PROGRAM P_Prog2
VAR

	fbKL6401 					: FB_LON_KL6401;

	fbREAD_032		: FB_READ_032_SNVT_res_kilo;
	fbSEND_032		: FB_SEND_032_SNVT_res_kilo;

	fbREAD_033		: FB_READ_033_SNVT_sound_db;
	fbSEND_033		: FB_SEND_033_SNVT_sound_db;

	fbREAD_034		: FB_READ_034_SNVT_speed;
	fbSEND_034		: FB_SEND_034_SNVT_speed;

	fbREAD_035		: FB_READ_035_SNVT_speed_mil;
	fbSEND_035		: FB_SEND_035_SNVT_speed_mil;

	fbREAD_036		: FB_READ_036_SNVT_str_asc;
	fbSEND_036		: FB_SEND_036_SNVT_str_asc;

	fbREAD_037		: FB_READ_037_SNVT_str_int;
	fbSEND_037		: FB_SEND_037_SNVT_str_int;

	fbREAD_038		: FB_READ_038_SNVT_telcom;
	fbSEND_038		: FB_SEND_038_SNVT_telcom;

	fbREAD_039		: FB_READ_039_SNVT_temp;
	fbSEND_039		: FB_SEND_039_SNVT_temp;
(*
	fbREAD_040		: FB_READ_040;
	fbSEND_040		: FB_SEND_008_SNVT_count;
*)
	fbREAD_041		: FB_READ_041_SNVT_vol;
	fbSEND_041		: FB_SEND_041_SNVT_vol;

	fbREAD_042		: FB_READ_042_SNVT_vol_kilo;
	fbSEND_042		: FB_SEND_042_SNVT_vol_kilo;

	fbREAD_043		: FB_READ_043_SNVT_vol_mil;
	fbSEND_043		: FB_SEND_043_SNVT_vol_mil;

	fbREAD_044		: FB_READ_044_SNVT_volt;
	fbSEND_044		: FB_SEND_044_SNVT_volt;

	fbREAD_045		: FB_READ_045_SNVT_volt_dbmv;
	fbSEND_045		: FB_SEND_045_SNVT_volt_dbmv;

	fbREAD_046		: FB_READ_046_SNVT_volt_kilo;
	fbSEND_046		: FB_SEND_046_SNVT_volt_kilo;

	fbREAD_047		: FB_READ_047_SNVT_volt_mil;
	fbSEND_047		: FB_SEND_047_SNVT_volt_mil;

	fbREAD_048		: FB_READ_048_SNVT_amp_f;
	fbSEND_048		: FB_SEND_048_SNVT_amp_f;

	fbREAD_049		: FB_READ_049_SNVT_angle_f;
	fbSEND_049		: FB_SEND_049_SNVT_angle_f;

	fbREAD_050		: FB_READ_050_SNVT_angle_vel_f;
	fbSEND_050		: FB_SEND_050_SNVT_angle_vel_f;

	fbREAD_051		: FB_READ_051_SNVT_count_f;
	fbSEND_051		: FB_SEND_051_SNVT_count_f;

	fbREAD_052		: FB_READ_052_SNVT_count_inc_f;
	fbSEND_052		: FB_SEND_052_SNVT_count_inc_f;

	fbREAD_053		: FB_READ_053_SNVT_flow_f;
	fbSEND_053		: FB_SEND_053_SNVT_flow_f;

	fbREAD_054		: FB_READ_054_SNVT_length_f;
	fbSEND_054		: FB_SEND_054_SNVT_length_f;

	fbREAD_055		: FB_READ_055_SNVT_lev_cont_f;
	fbSEND_055		: FB_SEND_055_SNVT_lev_cont_f;

	fbREAD_056		: FB_READ_056_SNVT_mass_f;
	fbSEND_056		: FB_SEND_056_SNVT_mass_f;

	fbREAD_057		: FB_READ_057_SNVT_power_f;
	fbSEND_057		: FB_SEND_057_SNVT_power_f;

	fbREAD_058		: FB_READ_058_SNVT_ppm_f;
	fbSEND_058		: FB_SEND_058_SNVT_ppm_f;

	fbREAD_059		: FB_READ_059_SNVT_press_f;
	fbSEND_059		: FB_SEND_059_SNVT_press_f;

	fbREAD_060		: FB_READ_060_SNVT_res_f;
	fbSEND_060		: FB_SEND_060_SNVT_res_f;

	fbREAD_061		: FB_READ_061_SNVT_sound_db_f;
	fbSEND_061		: FB_SEND_061_SNVT_sound_db_f;

	fbREAD_062		: FB_READ_062_SNVT_speed_f;
	fbSEND_062		: FB_SEND_062_SNVT_speed_f;

END_VAR

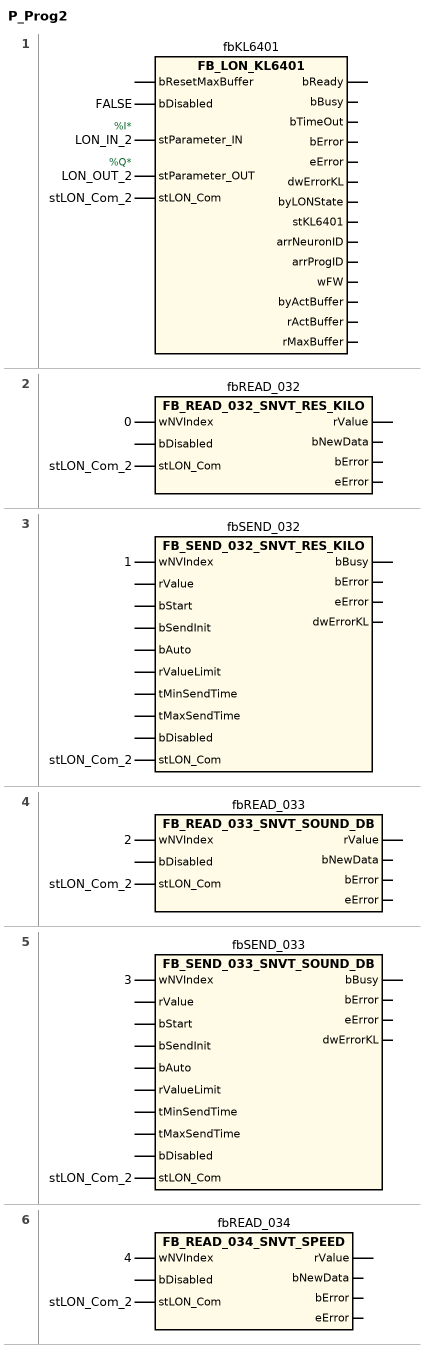
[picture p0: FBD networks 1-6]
// NETWORK 1
//   LON_IN_2: AT %I*
//   LON_OUT_2: AT %Q*
fbKL6401(
    bDisabled := FALSE,
    stParameter_IN := LON_IN_2,
    stParameter_OUT := LON_OUT_2,
    stLON_Com := stLON_Com_2); // FB_LON_KL6401

// NETWORK 2
fbREAD_032(wNVIndex := 0, stLON_Com := stLON_Com_2); // FB_READ_032_SNVT_RES_KILO

// NETWORK 3
fbSEND_032(wNVIndex := 1, stLON_Com := stLON_Com_2); // FB_SEND_032_SNVT_RES_KILO

// NETWORK 4
fbREAD_033(wNVIndex := 2, stLON_Com := stLON_Com_2); // FB_READ_033_SNVT_SOUND_DB

// NETWORK 5
fbSEND_033(wNVIndex := 3, stLON_Com := stLON_Com_2); // FB_SEND_033_SNVT_SOUND_DB

// NETWORK 6
fbREAD_034(wNVIndex := 4, stLON_Com := stLON_Com_2); // FB_READ_034_SNVT_SPEED

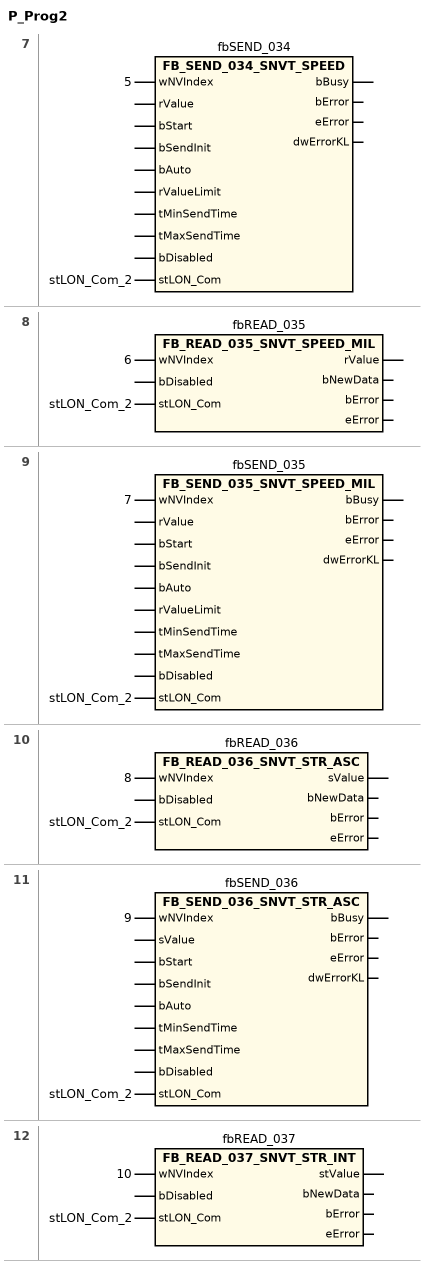
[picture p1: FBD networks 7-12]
// NETWORK 7
fbSEND_034(wNVIndex := 5, stLON_Com := stLON_Com_2); // FB_SEND_034_SNVT_SPEED

// NETWORK 8
fbREAD_035(wNVIndex := 6, stLON_Com := stLON_Com_2); // FB_READ_035_SNVT_SPEED_MIL

// NETWORK 9
fbSEND_035(wNVIndex := 7, stLON_Com := stLON_Com_2); // FB_SEND_035_SNVT_SPEED_MIL

// NETWORK 10
fbREAD_036(wNVIndex := 8, stLON_Com := stLON_Com_2); // FB_READ_036_SNVT_STR_ASC

// NETWORK 11
fbSEND_036(wNVIndex := 9, stLON_Com := stLON_Com_2); // FB_SEND_036_SNVT_STR_ASC

// NETWORK 12
fbREAD_037(wNVIndex := 10, stLON_Com := stLON_Com_2); // FB_READ_037_SNVT_STR_INT

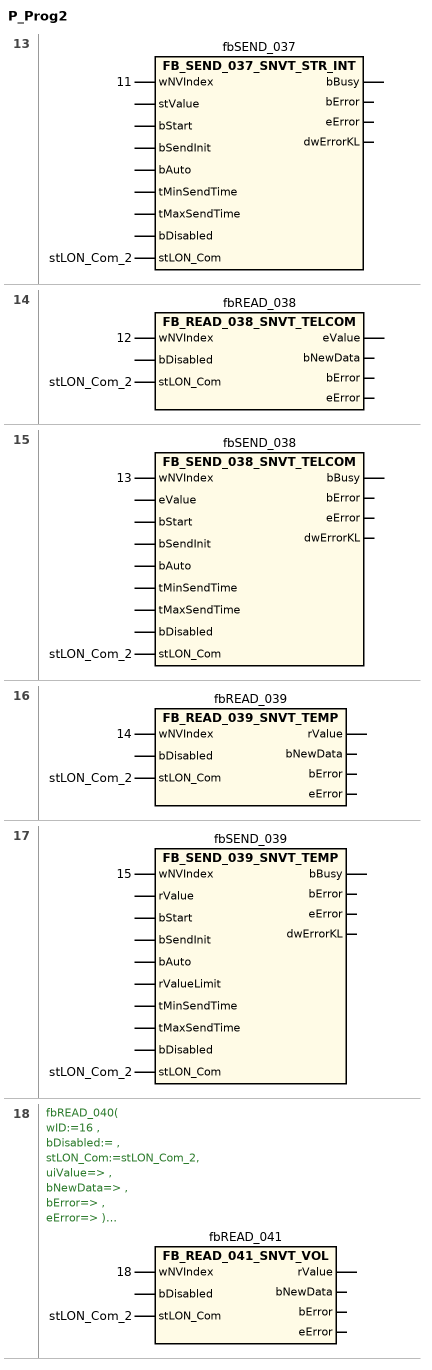
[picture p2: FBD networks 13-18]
// NETWORK 13
fbSEND_037(wNVIndex := 11, stLON_Com := stLON_Com_2); // FB_SEND_037_SNVT_STR_INT

// NETWORK 14
fbREAD_038(wNVIndex := 12, stLON_Com := stLON_Com_2); // FB_READ_038_SNVT_TELCOM

// NETWORK 15
fbSEND_038(wNVIndex := 13, stLON_Com := stLON_Com_2); // FB_SEND_038_SNVT_TELCOM

// NETWORK 16
fbREAD_039(wNVIndex := 14, stLON_Com := stLON_Com_2); // FB_READ_039_SNVT_TEMP

// NETWORK 17
fbSEND_039(wNVIndex := 15, stLON_Com := stLON_Com_2); // FB_SEND_039_SNVT_TEMP

// NETWORK 18
//
//
// fbREAD_040(
// 	wID:=16 ,
// 	bDisabled:= ,
// 	stLON_Com:=stLON_Com_2,
// 	uiValue=> ,
// 	bNewData=> ,
// 	bError=> ,
// 	eError=> );
// fbREAD_040.uiValue;
// fbREAD_040.bError;
// fbREAD_040.eError;
//
// fbSEND_040(
// 	wID:=17 ,
// 	bStart:= ,
// 	uiValue:= ,
// 	bDisabled:= ,
// 	stLON_Com:=stLON_Com_2,
// 	bError=> ,
// 	eError=> );
// fbSEND_040.uiValue;
// fbSEND_040.bStart;
// fbSEND_040.bError;
// fbSEND_040.eError;
//
//
//
//   fbREAD_041: fbREAD_040 : FB_READ_040; fbSEND_040 : FB_SEND_008_SNVT_count;
fbREAD_041(wNVIndex := 18, stLON_Com := stLON_Com_2); // FB_READ_041_SNVT_VOL

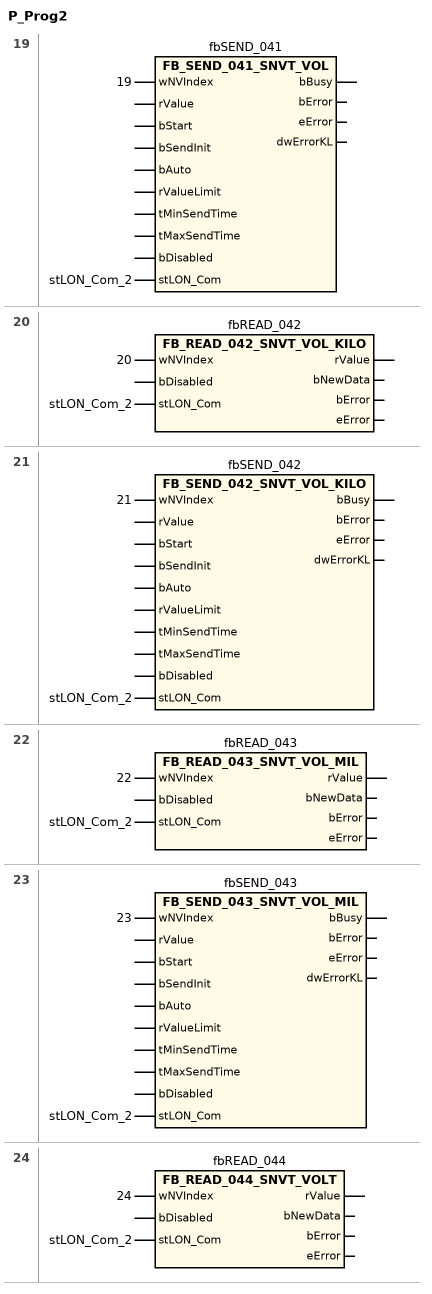
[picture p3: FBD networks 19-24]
// NETWORK 19
fbSEND_041(wNVIndex := 19, stLON_Com := stLON_Com_2); // FB_SEND_041_SNVT_VOL

// NETWORK 20
fbREAD_042(wNVIndex := 20, stLON_Com := stLON_Com_2); // FB_READ_042_SNVT_VOL_KILO

// NETWORK 21
fbSEND_042(wNVIndex := 21, stLON_Com := stLON_Com_2); // FB_SEND_042_SNVT_VOL_KILO

// NETWORK 22
fbREAD_043(wNVIndex := 22, stLON_Com := stLON_Com_2); // FB_READ_043_SNVT_VOL_MIL

// NETWORK 23
fbSEND_043(wNVIndex := 23, stLON_Com := stLON_Com_2); // FB_SEND_043_SNVT_VOL_MIL

// NETWORK 24
fbREAD_044(wNVIndex := 24, stLON_Com := stLON_Com_2); // FB_READ_044_SNVT_VOLT

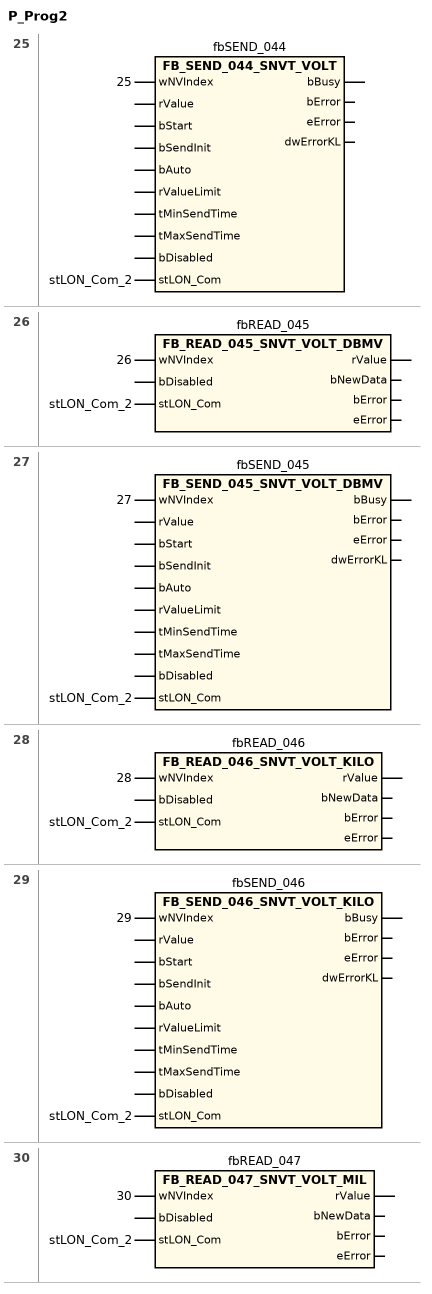
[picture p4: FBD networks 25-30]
// NETWORK 25
fbSEND_044(wNVIndex := 25, stLON_Com := stLON_Com_2); // FB_SEND_044_SNVT_VOLT

// NETWORK 26
fbREAD_045(wNVIndex := 26, stLON_Com := stLON_Com_2); // FB_READ_045_SNVT_VOLT_DBMV

// NETWORK 27
fbSEND_045(wNVIndex := 27, stLON_Com := stLON_Com_2); // FB_SEND_045_SNVT_VOLT_DBMV

// NETWORK 28
fbREAD_046(wNVIndex := 28, stLON_Com := stLON_Com_2); // FB_READ_046_SNVT_VOLT_KILO

// NETWORK 29
fbSEND_046(wNVIndex := 29, stLON_Com := stLON_Com_2); // FB_SEND_046_SNVT_VOLT_KILO

// NETWORK 30
fbREAD_047(wNVIndex := 30, stLON_Com := stLON_Com_2); // FB_READ_047_SNVT_VOLT_MIL

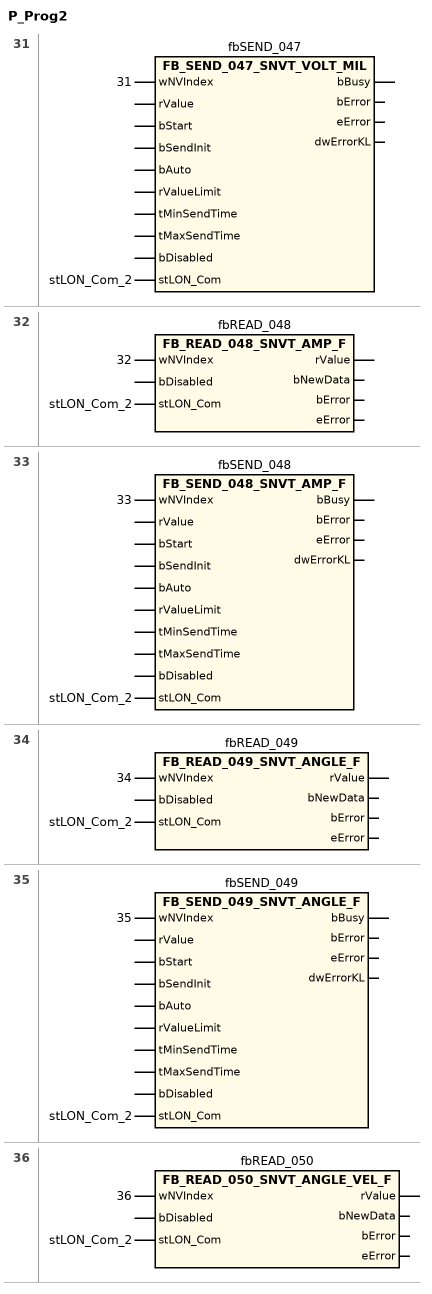
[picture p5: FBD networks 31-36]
// NETWORK 31
fbSEND_047(wNVIndex := 31, stLON_Com := stLON_Com_2); // FB_SEND_047_SNVT_VOLT_MIL

// NETWORK 32
fbREAD_048(wNVIndex := 32, stLON_Com := stLON_Com_2); // FB_READ_048_SNVT_AMP_F

// NETWORK 33
fbSEND_048(wNVIndex := 33, stLON_Com := stLON_Com_2); // FB_SEND_048_SNVT_AMP_F

// NETWORK 34
fbREAD_049(wNVIndex := 34, stLON_Com := stLON_Com_2); // FB_READ_049_SNVT_ANGLE_F

// NETWORK 35
fbSEND_049(wNVIndex := 35, stLON_Com := stLON_Com_2); // FB_SEND_049_SNVT_ANGLE_F

// NETWORK 36
fbREAD_050(wNVIndex := 36, stLON_Com := stLON_Com_2); // FB_READ_050_SNVT_ANGLE_VEL_F

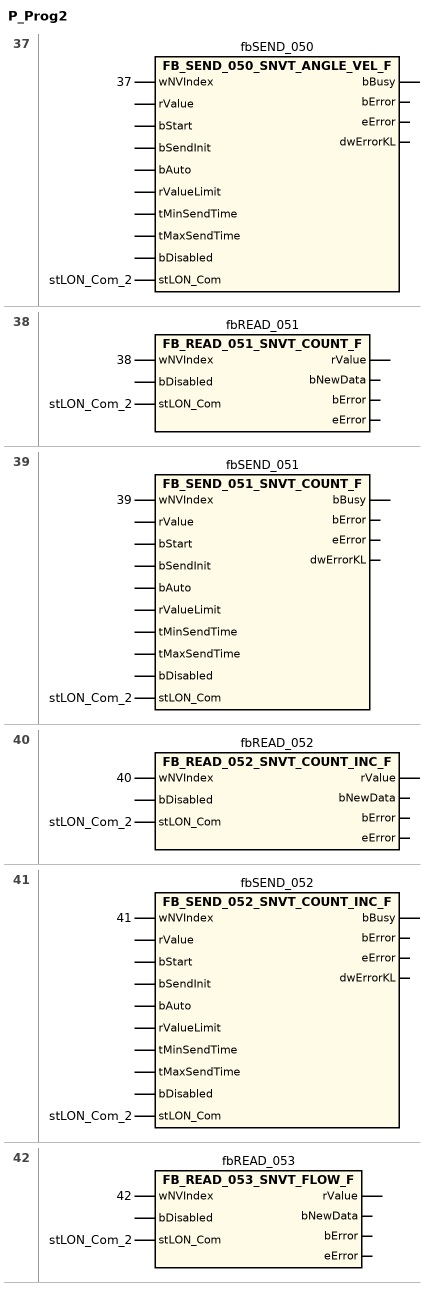
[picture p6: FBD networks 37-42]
// NETWORK 37
fbSEND_050(wNVIndex := 37, stLON_Com := stLON_Com_2); // FB_SEND_050_SNVT_ANGLE_VEL_F

// NETWORK 38
fbREAD_051(wNVIndex := 38, stLON_Com := stLON_Com_2); // FB_READ_051_SNVT_COUNT_F

// NETWORK 39
fbSEND_051(wNVIndex := 39, stLON_Com := stLON_Com_2); // FB_SEND_051_SNVT_COUNT_F

// NETWORK 40
fbREAD_052(wNVIndex := 40, stLON_Com := stLON_Com_2); // FB_READ_052_SNVT_COUNT_INC_F

// NETWORK 41
fbSEND_052(wNVIndex := 41, stLON_Com := stLON_Com_2); // FB_SEND_052_SNVT_COUNT_INC_F

// NETWORK 42
fbREAD_053(wNVIndex := 42, stLON_Com := stLON_Com_2); // FB_READ_053_SNVT_FLOW_F

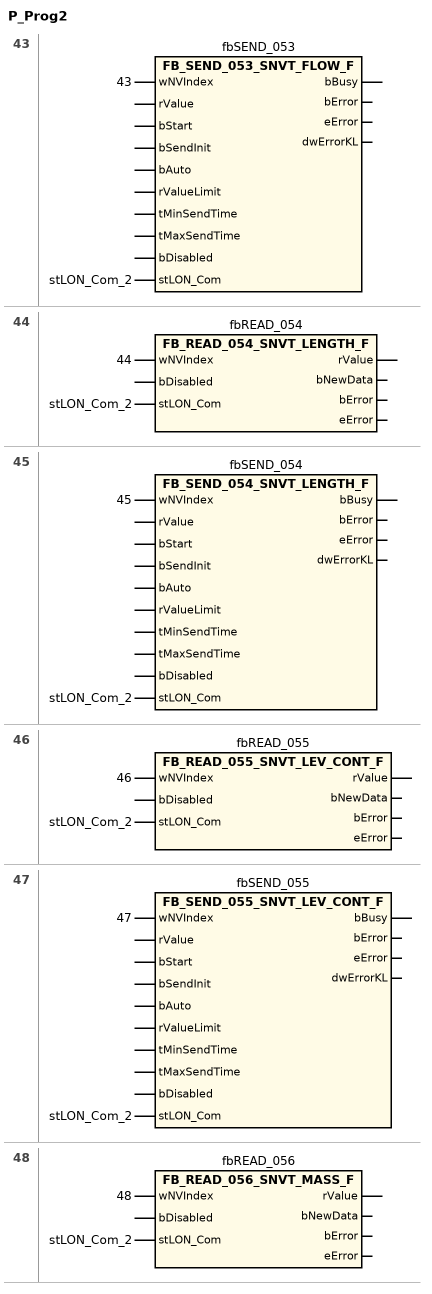
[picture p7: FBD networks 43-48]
// NETWORK 43
fbSEND_053(wNVIndex := 43, stLON_Com := stLON_Com_2); // FB_SEND_053_SNVT_FLOW_F

// NETWORK 44
fbREAD_054(wNVIndex := 44, stLON_Com := stLON_Com_2); // FB_READ_054_SNVT_LENGTH_F

// NETWORK 45
fbSEND_054(wNVIndex := 45, stLON_Com := stLON_Com_2); // FB_SEND_054_SNVT_LENGTH_F

// NETWORK 46
fbREAD_055(wNVIndex := 46, stLON_Com := stLON_Com_2); // FB_READ_055_SNVT_LEV_CONT_F

// NETWORK 47
fbSEND_055(wNVIndex := 47, stLON_Com := stLON_Com_2); // FB_SEND_055_SNVT_LEV_CONT_F

// NETWORK 48
fbREAD_056(wNVIndex := 48, stLON_Com := stLON_Com_2); // FB_READ_056_SNVT_MASS_F

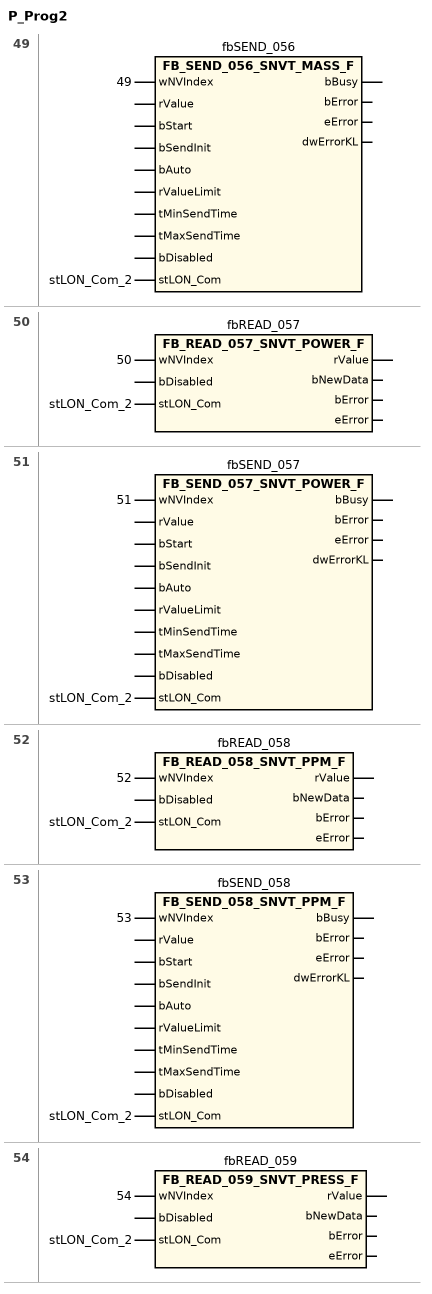
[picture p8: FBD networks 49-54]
// NETWORK 49
fbSEND_056(wNVIndex := 49, stLON_Com := stLON_Com_2); // FB_SEND_056_SNVT_MASS_F

// NETWORK 50
fbREAD_057(wNVIndex := 50, stLON_Com := stLON_Com_2); // FB_READ_057_SNVT_POWER_F

// NETWORK 51
fbSEND_057(wNVIndex := 51, stLON_Com := stLON_Com_2); // FB_SEND_057_SNVT_POWER_F

// NETWORK 52
fbREAD_058(wNVIndex := 52, stLON_Com := stLON_Com_2); // FB_READ_058_SNVT_PPM_F

// NETWORK 53
fbSEND_058(wNVIndex := 53, stLON_Com := stLON_Com_2); // FB_SEND_058_SNVT_PPM_F

// NETWORK 54
fbREAD_059(wNVIndex := 54, stLON_Com := stLON_Com_2); // FB_READ_059_SNVT_PRESS_F

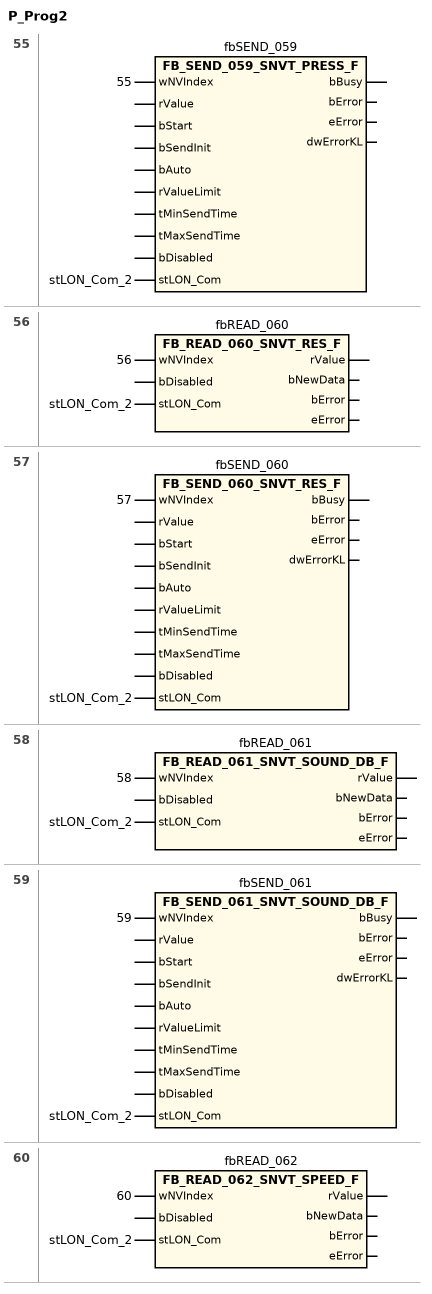
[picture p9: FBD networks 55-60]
// NETWORK 55
fbSEND_059(wNVIndex := 55, stLON_Com := stLON_Com_2); // FB_SEND_059_SNVT_PRESS_F

// NETWORK 56
fbREAD_060(wNVIndex := 56, stLON_Com := stLON_Com_2); // FB_READ_060_SNVT_RES_F

// NETWORK 57
fbSEND_060(wNVIndex := 57, stLON_Com := stLON_Com_2); // FB_SEND_060_SNVT_RES_F

// NETWORK 58
fbREAD_061(wNVIndex := 58, stLON_Com := stLON_Com_2); // FB_READ_061_SNVT_SOUND_DB_F

// NETWORK 59
fbSEND_061(wNVIndex := 59, stLON_Com := stLON_Com_2); // FB_SEND_061_SNVT_SOUND_DB_F

// NETWORK 60
fbREAD_062(wNVIndex := 60, stLON_Com := stLON_Com_2); // FB_READ_062_SNVT_SPEED_F

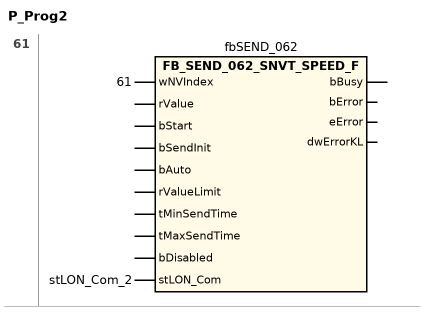
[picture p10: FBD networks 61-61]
// NETWORK 61
fbSEND_062(wNVIndex := 61, stLON_Com := stLON_Com_2); // FB_SEND_062_SNVT_SPEED_F

END_PROGRAM
